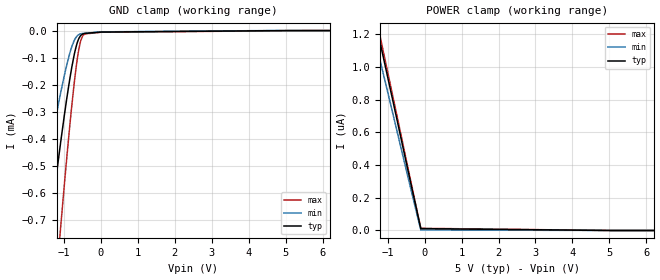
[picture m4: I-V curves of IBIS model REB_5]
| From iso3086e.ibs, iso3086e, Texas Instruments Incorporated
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|   REB_5 Model
[Model]   REB_5
Model_type   Input
Vinl   = 0.8
Vinh   = 2
|   typ   min   max
C_comp   5.76pF   5.75pF   5.79pF
[Voltage Range]   5   4.5   5.5
[Temperature Range]   40   125   -40
[Power Clamp Reference]   5   4.5   5.5
[GND Clamp Reference]   0   0   0
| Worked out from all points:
|   GND clamp passes 1 mA (typ) near -1.61 V on its own axis
[GND Clamp]
|   Voltage   I(typ)   I(min)   I(max)
-5V       -5.533mA   -3.836mA   -8.081mA
-1.782V   -1.206mA   -765.7uA   -1.924mA
-1.738V   -1.151mA   -728uA     -1.843mA
-1.43V    -786.8uA   -479.6uA   -1.299mA
-1.34V    -684.4uA   -410.6uA   -1.144mA
-1.107V   -432.5uA   -242.9uA   -757.2uA
-785mV    -134.1uA   -58.95uA   -274.8uA
-665mV    -56.86uA   -23.66uA   -131.3uA
-560mV    -20.64uA   -12.59uA   -45.53uA
-432.5mV  -10.46uA   -9.987uA   -12.44uA
2.5mV     -5.54uA    -4.744uA   -6.193uA
10V       0A         0A         0A
[POWER Clamp]
|   Voltage   I(typ)   I(min)   I(max)
-5V       5.139uA    4.686uA    5.292uA
-1.438V   1.388uA    1.257uA    1.432uA
-1.355V   1.303uA    1.18uA     1.345uA
-1.34V    1.288uA    1.166uA    1.329uA
-1.212V   1.156uA    1.046uA    1.194uA
-102.5mV  11.14nA    3.276nA    13.26nA
5.005V    0A         0A         0A
10V       0A         0A         0A
